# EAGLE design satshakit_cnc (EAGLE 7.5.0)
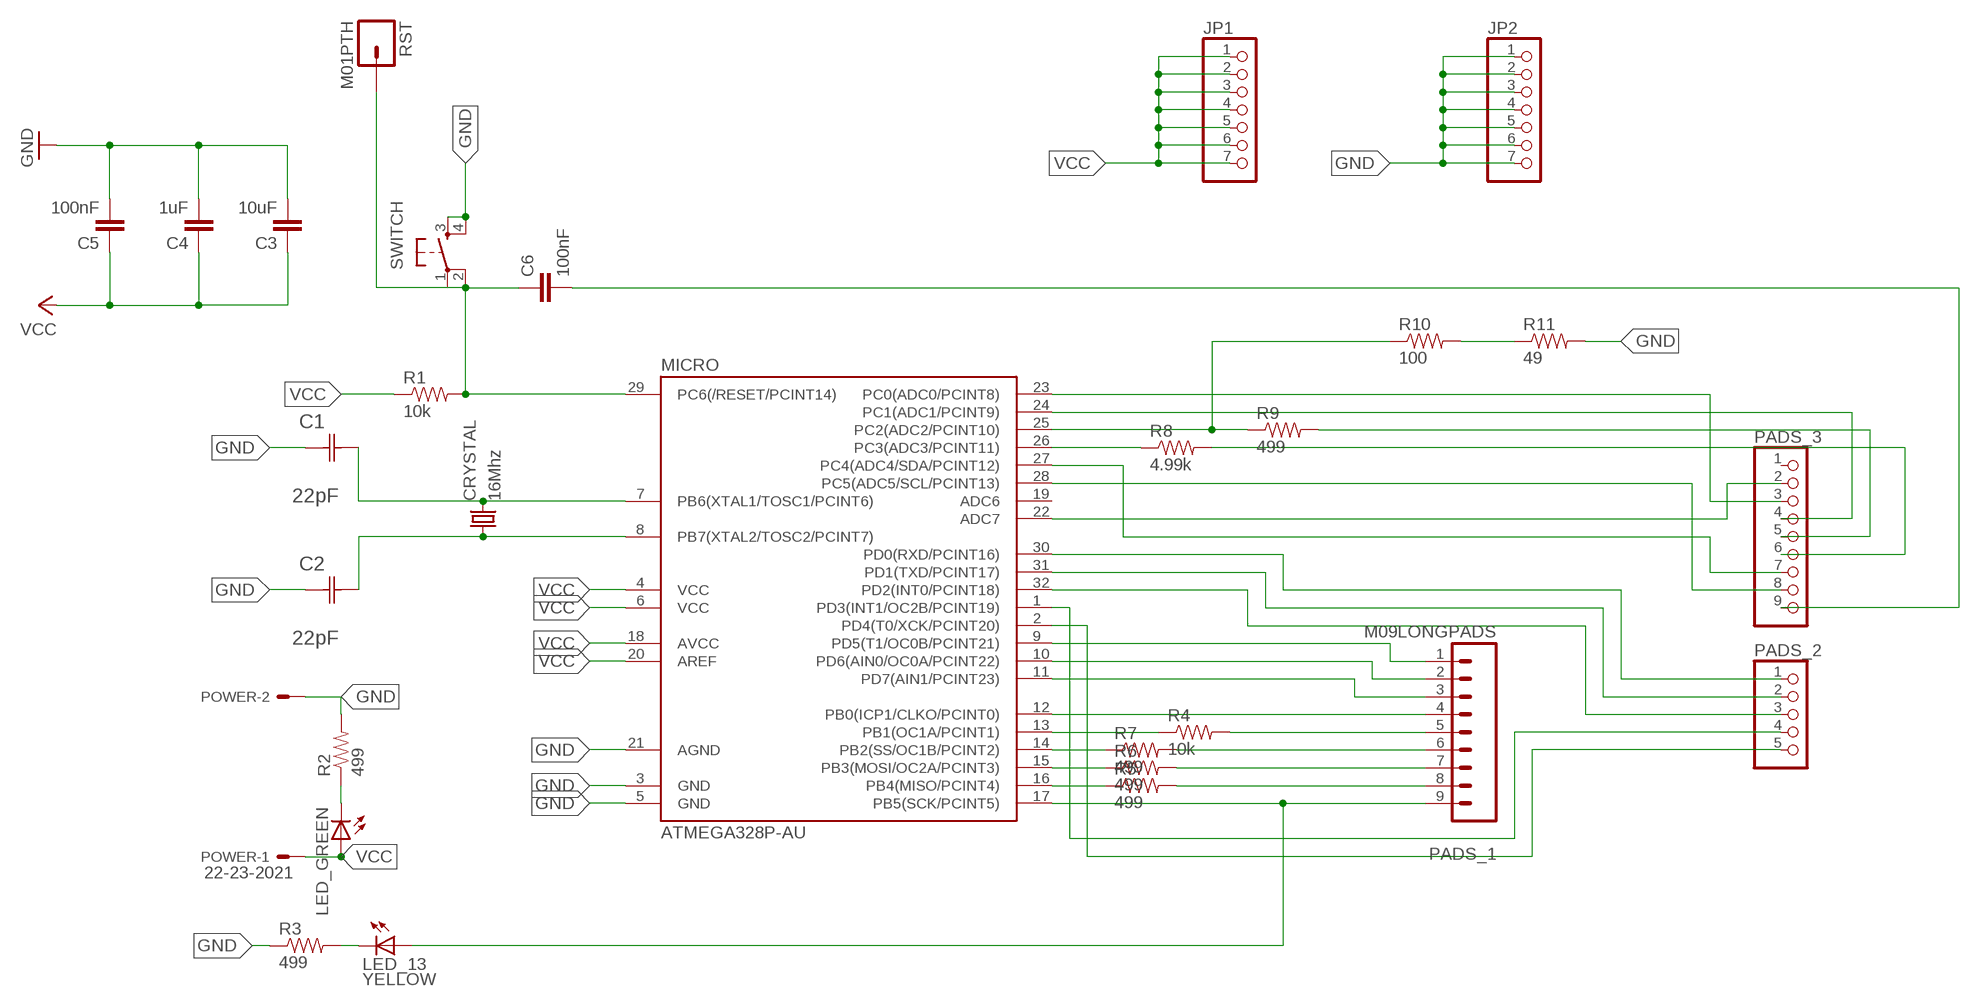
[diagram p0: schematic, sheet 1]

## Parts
C1  22pF  0612ZC225MAT2A  [CAPC3216X178N]
C2  22pF  0612ZC225MAT2A  [CAPC3216X178N]
C3  10uF  CAP1206  [1206]
C4  1uF  CAP1206  [1206]
C5  100nF  CAP1206  [1206]
C6  100nF  CAP1206  [1206]
CRYSTAL  16Mhz  CSM-7X-DU  [CSM-7X-DU]
JP1  PINHD-1X7  [1X07]
JP2  PINHD-1X7  [1X07]
LED_13  YELLOW  LED1206  [1206]
LED_GREEN  LED1206  [1206]
MICRO  ATMEGA328P-AU  ATMEGA48/88/168-AU  [TQFP32-08]
PADS_1  M09LONGPADS  [1X09_LONGPADS]
PADS_2  PINHD-1X5  [1X05]
PADS_3  PINHD-1X9  [1X09]
POWER  22-23-2021  [22-23-2021]
R1  10k  RESISTOR1206  [1206]
R2  499  RESISTOR1206  [1206]
R3  499  RESISTOR1206  [1206]
R4  10k  RESISTOR1206  [1206]
R5  499  RESISTOR1206  [1206]
R6  499  RESISTOR1206  [1206]
R7  499  RESISTOR1206  [1206]
R8  4.99k  RESISTOR1206  [1206]
R9  499  RESISTOR1206  [1206]
R10  100  RESISTOR1206  [1206]
R11  49  RESISTOR1206  [1206]
RST  M01PTH  [1X01]
SWITCH  6MM_SWITCH6MM_SWITCH  [6MM_SWITCH]

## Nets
GND: C1.1(C1) C2.1(C1) C3.2 C4.2 C5.2 JP2.1 JP2.2 JP2.3 JP2.4 JP2.5 JP2.6 JP2.7 MICRO.3(GND) MICRO.5(GND) MICRO.21(AGND) POWER.2 R2.2 R3.1 R11.2 SWITCH.3(S) SWITCH.4(S1)
N$1: MICRO.9(PD5(T1/OC0B/PCINT21)) PADS_1.1
N$2: C1.2(C2) CRYSTAL.2 MICRO.7(PB6(XTAL1/TOSC1/PCINT6))
N$3: C6.2 PADS_3.9
N$4: MICRO.10(PD6(AIN0/OC0A/PCINT22)) PADS_1.2
N$5: MICRO.11(PD7(AIN1/PCINT23)) PADS_1.3
N$6: MICRO.12(PB0(ICP1/CLKO/PCINT0)) PADS_1.4
N$7: MICRO.13(PB1(OC1A/PCINT1)) R4.1
N$8: MICRO.14(PB2(SS/OC1B/PCINT2)) R7.1
N$9: C2.2(C2) CRYSTAL.1 MICRO.8(PB7(XTAL2/TOSC2/PCINT7))
N$10: MICRO.15(PB3(MOSI/OC2A/PCINT3)) R6.1
N$11: MICRO.16(PB4(MISO/PCINT4)) R5.1
N$12: LED_13.1(A) MICRO.17(PB5(SCK/PCINT5)) PADS_1.9
N$13: PADS_1.6 R7.2
N$14: MICRO.22(ADC7) PADS_3.2
N$15: MICRO.23(PC0(ADC0/PCINT8)) PADS_3.3
N$16: MICRO.24(PC1(ADC1/PCINT9)) PADS_3.4
N$17: PADS_3.5 R9.2
N$18: PADS_3.6 R8.2
N$19: MICRO.27(PC4(ADC4/SDA/PCINT12)) PADS_3.7
N$20: MICRO.30(PD0(RXD/PCINT16)) PADS_2.1
N$21: MICRO.31(PD1(TXD/PCINT17)) PADS_2.2
N$22: MICRO.32(PD2(INT0/PCINT18)) PADS_2.3
N$23: MICRO.1(PD3(INT1/OC2B/PCINT19)) PADS_2.4
N$24: MICRO.2(PD4(T0/XCK/PCINT20)) PADS_2.5
N$25: MICRO.28(PC5(ADC5/SCL/PCINT13)) PADS_3.8
N$26: LED_GREEN.2(C) R2.1
N$27: LED_13.2(C) R3.2
N$28: C6.1 MICRO.29(PC6(/RESET/PCINT14)) R1.2 RST.1 SWITCH.1(P) SWITCH.2(P1)
N$30: PADS_1.7 R6.2
N$31: PADS_1.8 R5.2
N$32: PADS_1.5 R4.2
N$33: MICRO.26(PC3(ADC3/PCINT11)) R8.1
N$34: MICRO.25(PC2(ADC2/PCINT10)) R9.1 R10.1
N$35: R10.2 R11.1
VCC: C3.1 C4.1 C5.1 JP1.1 JP1.2 JP1.3 JP1.4 JP1.5 JP1.6 JP1.7 LED_GREEN.1(A) MICRO.4(VCC) MICRO.6(VCC) MICRO.18(AVCC) MICRO.20(AREF) POWER.1 R1.1
Unconnected: MICRO.19(ADC6) PADS_3.1

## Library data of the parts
C1 C2 = AVX_By_element14_Batch_1:0612ZC225MAT2A: Capacitor 1206; MPN: 0612ZC225MAT2A; OC_FARNELL: -; OC_NEWARK: 12N3209; SUPPLIER: AVX; TOLERANCE: ±20%; VALUE: 2.2µF; VOLTAGERATING: 10V
C3-C6 = 01_SparkFun:CAP: Capacitor
CRYSTAL = 01_FAB_Hello:CSM-7X-DU: SMD CRYSTAL; OC_FARNELL: unknown; OC_NEWARK: unknown
JP1 JP2 = pinhead:PINHD-1X7: PIN HEADER
LED_13 LED_GREEN = 01_FAB_Hello:LED
MICRO = atmega8:ATMEGA48/88/168
PADS_1 = 01_SparkFun:M09: Header 9 Standard 9-pin 0.1" header. Use with straight break away headers (SKU : PRT-00116), right angle break away headers (PRT-00553), swiss pins (PRT-00743), machine pins (PRT-00117), and female headers (PRT-00115).
PADS_2 = pinhead:PINHD-1X5: PIN HEADER
PADS_3 = pinhead:PINHD-1X9: PIN HEADER
POWER = con-molex:22-23-2021: .100" (2.54mm) Center Header - 2 Pin; MF: MOLEX; MPN: 22-23-2021; OC_FARNELL: 1462926; OC_NEWARK: 25C3832
R1-R11 = 01_SparkFun:RESISTOR: Resistor
RST = 01_SparkFun:M01: Header 1
SWITCH = 01_FAB_Hello:6MM_SWITCH: OMRON SWITCH

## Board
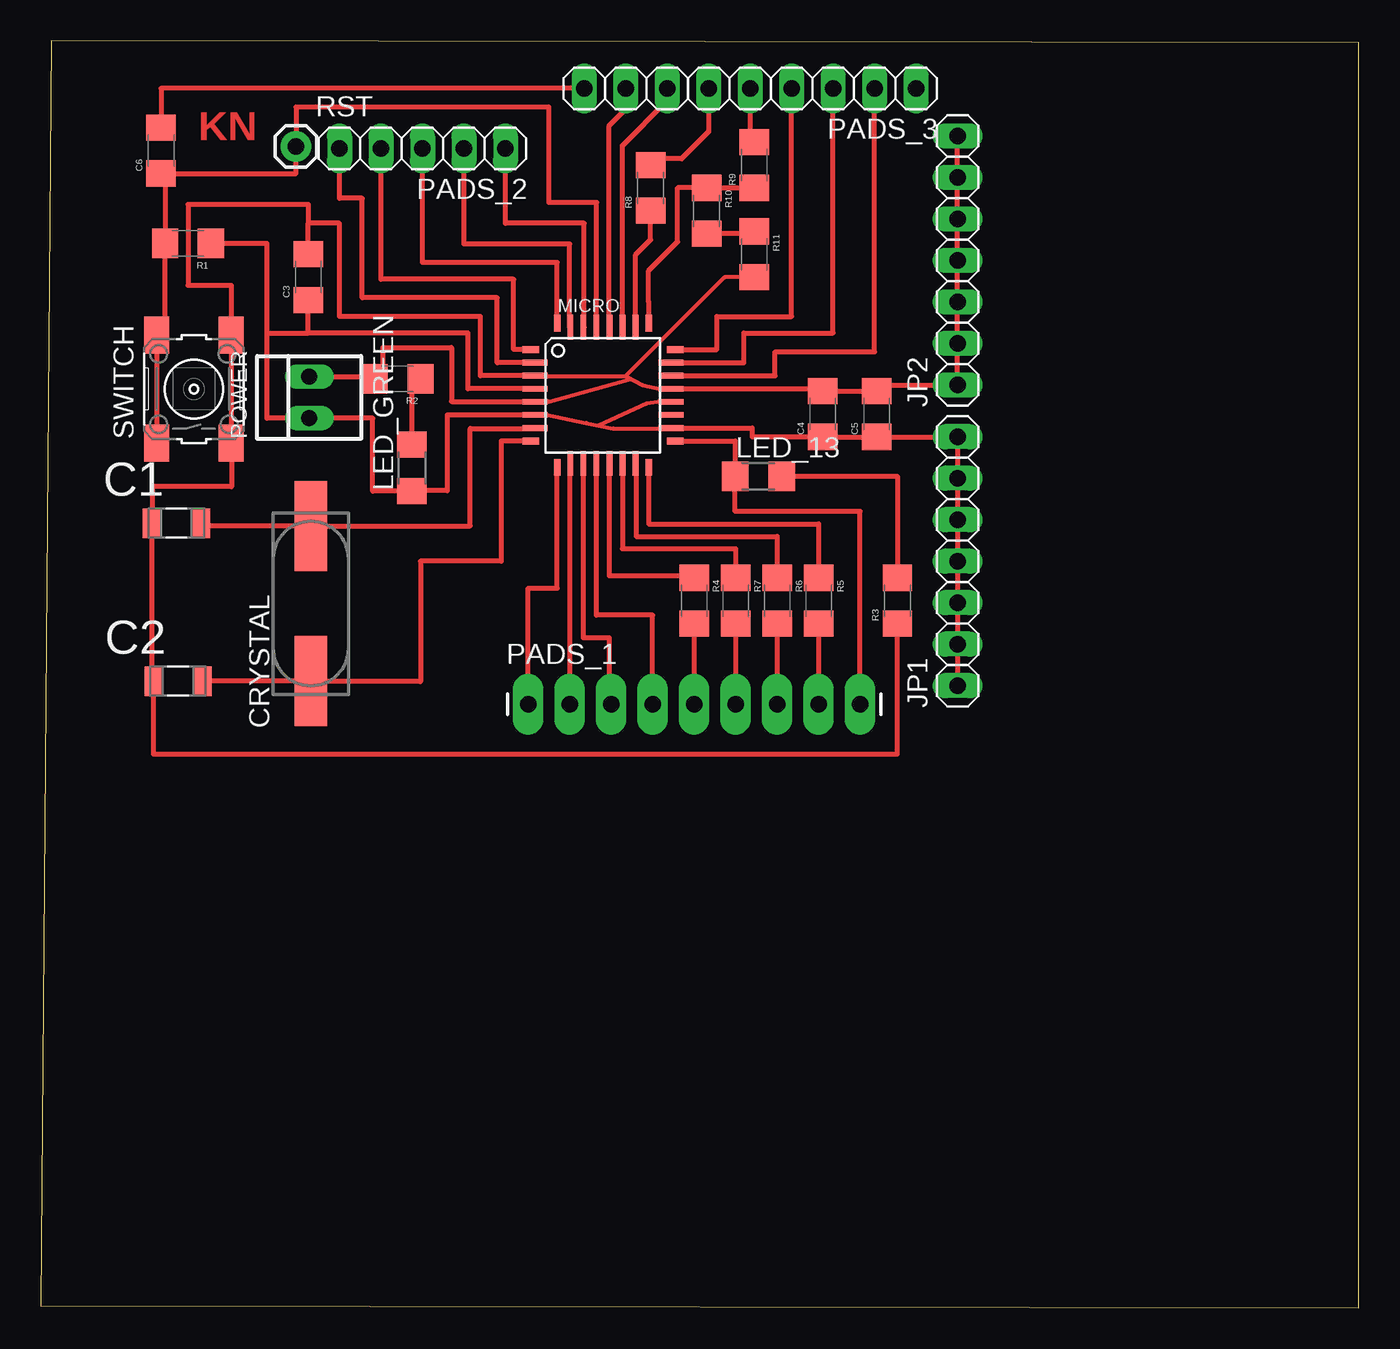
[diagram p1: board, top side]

Size 80.7 x 77.59 mm. Coordinates in mm from the lower left corner, seen from the top.
Outline: 0,0.13 80.7,0 80.7,77.46 0.63,77.59 0,0.13
Copper layers (1*16): Top 0.035mm / dielectric 1.5mm / Bottom 0.035mm
Design rules "default": minimum track width 10mil, minimum drill 24mil, track to track 8mil, track to pad 8mil, pad to pad 8mil, via to via 8mil, smd to smd 8mil, copper to edge 40mil, drill to drill 8mil, minimum pad ring 10mil, minimum via ring 8mil, stop-mask expansion 4mil, vias tented up to drill 0mil, thermal gap 10mil

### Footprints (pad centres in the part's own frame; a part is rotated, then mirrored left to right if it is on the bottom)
CAPC3216X178N = smd 1.118 x 1.803: 1 -1.499,0; 2 1.499,0
1206 = smd 1.6 x 1.8: 1 -1.4,0; 2 1.4,0
CSM-7X-DU = smd 5.5 x 2: 1 -4.75,0; 2 4.75,0
1X07 = drill 1.016 long: 1 -7.62,0; 2 -5.08,0; 3 -2.54,0; 4 0,0; 5 2.54,0; 6 5.08,0; 7 7.62,0
1206' = smd 1.6 x 1.803: 1 -1.422,0; 2 1.422,0
TQFP32-08 = smd 1.016 x 0.406: 1 -4.42,2.8; 8 -4.42,-2.8; 17 4.42,-2.8; 24 4.42,2.8 | smd 1.524 x 0.356: 2 -4.166,2; 3 -4.166,1.2; 4 -4.166,0.4; 5 -4.166,-0.4; 6 -4.166,-1.2; 7 -4.166,-2; 18 4.166,-2; 19 4.166,-1.2; 20 4.166,-0.4; 21 4.166,0.4; 22 4.166,1.2; 23 4.166,2 | smd 0.406 x 1.016: 9 -2.8,-4.42; 16 2.8,-4.42; 25 2.8,4.42; 32 -2.8,4.42 | smd 0.356 x 1.524: 10 -2,-4.166; 11 -1.2,-4.166; 12 -0.4,-4.166; 13 0.4,-4.166; 14 1.2,-4.166; 15 2,-4.166; 26 2,4.166; 27 1.2,4.166; 28 0.4,4.166; 29 -0.4,4.166; 30 -1.2,4.166; 31 -2,4.166
1X09_LONGPADS = drill 1.016 pad 1.88 long: 1 0,0; 2 2.54,0; 3 5.08,0; 4 7.62,0; 5 10.16,0; 6 12.7,0; 7 15.24,0; 8 17.78,0; 9 20.32,0
1X05 = drill 1.016 long: 1 -5.08,0; 2 -2.54,0; 3 0,0; 4 2.54,0; 5 5.08,0
1X09 = drill 1.016 long: 1 -10.16,0; 2 -7.62,0; 3 -5.08,0; 4 -2.54,0; 5 0,0; 6 2.54,0; 7 5.08,0; 8 7.62,0; 9 10.16,0
22-23-2021 = drill 1 long: 1 -1.27,0; 2 1.27,0
1X01 = drill 1.016 pad 1.88: 1 0,0
6MM_SWITCH = smd 2.286 x 1.524: 1 -3.302,2.286; 2 3.302,2.286; 3 -3.302,-2.286; 4 3.302,-2.286

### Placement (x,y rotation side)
C1  8.31,48.06 0 top
C2  8.41,38.38 0 top
C3  16.38,63.12 90 top
C4  47.88,54.74 90 top
C5  51.18,54.74 90 top
C6  7.37,70.87 90 top
CRYSTAL  16.54,43.13 90 top
JP1  56.13,45.72 90 top
JP2  56.13,64.14 90 top
LED_13  YELLOW  [1206']  43.94,50.93 0 top
LED_GREEN  [1206']  22.73,51.44 90 top
MICRO  34.42,55.88 0 top
PADS_1  29.84,36.96 0 top
PADS_2  23.37,70.99 180 top
PADS_3  43.43,74.68 180 top
POWER  16.43,55.75 90 top
R1  9.02,65.18 180 top
R2  21.84,56.9 180 top
R3  52.45,43.31 90 top
R4  40.01,43.31 270 top
R5  47.62,43.31 270 top
R6  45.09,43.31 270 top
R7  42.55,43.31 270 top
R8  37.34,68.58 90 top
R9  43.69,69.98 90 top
R10  40.77,67.18 270 top
R11  43.69,64.52 270 top
RST  15.62,71.12 0 top
SWITCH  9.37,56.26 90 top

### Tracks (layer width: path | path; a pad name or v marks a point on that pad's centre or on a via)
GND
  Top 0.254: MICRO.3 30.28,57.05 35.8,57.05 | 35.8,57.05 36.83,56.52 37.97,56.26 | 30.86,55.5 31.12,55.5 35.99,56.84 | 35.99,56.84 36.13,56.88 | 35.8,57.05 35.99,56.84 | 35.8,57.05 41.87,63.12 R11.2
  Top 0.305: MICRO.5 | MICRO.21 | C1.1 6.81,38.38 C2.1 6.91,33.91 52.45,33.91 R3.1 | C1.1 6.73,48.06 | MICRO.5 30.25,55.5 25.15,55.5 25.15,58.8 20.95,58.8 20.95,56.77 R2.2 20.95,57.02 POWER.2 | C1.1 6.86,48.06 6.86,50.29 11.68,50.29 11.68,52.96 | MICRO.21 47.88,56.28 C4.2 C5.2 | 30.86,55.5 MICRO.5 | MICRO.21 37.97,56.26 | MICRO.3 26.92,57.08 26.92,60.71 18.29,60.71 18.29,66.42 16.38,66.42 | C3.2 16.38,66.42 | SWITCH.3 11.68,52.96 | 11.68,52.96 11.68,58.93 11.66,58.93 SWITCH.4 11.68,59.56 11.68,62.61 9.02,62.61 9.02,67.56 16.38,67.56 16.38,66.42 | 51.18,56.52 JP2.1 JP2.2 JP2.3 JP2.4 JP2.5 JP2.6 JP2.7
  Top 0.406: 51.18,56.52 C5.2
N$1
  Top 0.305: PADS_1.1 29.84,44.07 31.62,44.07 MICRO.9
N$2
  Top 0.305: 9.8,47.88 C1.2 9.8,47.88 | MICRO.7 30.25,53.85 26.29,53.85 26.29,47.88 CRYSTAL.2 9.8,47.88
N$3
  Top 0.305: PADS_3.9 7.37,74.68 C6.2
N$4
  Top 0.305: PADS_1.2 32.42,40.51 MICRO.10
N$5
  Top 0.305: MICRO.11 33.22,41.02 34.8,41.02 34.8,37.59 34.92,37.59 PADS_1.3
N$6
  Top 0.305: 34.04,51.71 MICRO.12 34.02,42.42 37.46,42.42 PADS_1.4
N$7
  Top 0.305: MICRO.13 34.8,51.71 34.8,44.83 40.01,44.83 R4.1
N$8
  Top 0.305: MICRO.14 35.62,46.48 42.55,46.48 R7.1
N$9
  Top 0.305: 9.91,38.35 C2.2 | MICRO.8 28.19,53.09 28.19,45.72 23.24,45.72 23.24,38.35 16.54,38.35 CRYSTAL.1 C2.2 | C2.2
N$10
  Top 0.305: MICRO.15 36.45,51.71 36.45,47.24 45.09,47.24 R6.1
N$11
  Top 0.305: MICRO.16 37.21,48.01 47.62,48.01 R5.1
N$12
  Top 0.305: PADS_1.9 50.16,48.77 42.52,48.77 LED_13.1 42.52,53.08 MICRO.17
N$13
  Top 0.305: R7.2 PADS_1.6
N$14
  Top 0.305: MICRO.22 44.96,57.08 44.96,58.55 51.05,58.55 PADS_3.2
N$15
  Top 0.305: MICRO.23 43.05,57.88 43.05,59.69 48.51,59.69 PADS_3.3
N$16
  Top 0.305: MICRO.24 41.4,58.68 41.4,60.71 45.97,60.71 PADS_3.4
N$17
  Top 0.305: PADS_3.5 43.43,71.38 R9.2
N$18
  Top 0.305: PADS_3.6 40.89,72.01 39.24,70.36 37.72,70.36 R8.2
N$19
  Top 0.305: MICRO.27 35.62,71.18 38.35,73.91 PADS_3.7
N$20
  Top 0.305: MICRO.30 33.27,60.05 33.27,66.42 28.45,66.42 PADS_2.1
N$21
  Top 0.305: MICRO.31 32.38,60.05 32.38,65.15 25.91,65.15 PADS_2.2
N$22
  Top 0.305: MICRO.32 31.62,64.01 23.37,64.01 PADS_2.3
N$23
  Top 0.305: MICRO.1 28.96,58.68 28.96,62.99 20.83,62.99 PADS_2.4
N$24
  Top 0.305: MICRO.2 27.94,57.88 27.94,61.85 19.69,61.85 19.69,67.94 18.29,67.94 PADS_2.5
N$25
  Top 0.305: MICRO.28 34.8,60.05 34.8,72.39 35.69,73.28 35.69,74.55 PADS_3.8
N$26
  Top 0.305: 23.62,56.64 R2.1 23.24,56.52 22.73,56.52 LED_GREEN.2
N$27
  Top 0.305: LED_13.2 52.45,50.93 R3.2
N$28
  Top 0.305: MICRO.29 34.04,60.05 34.04,67.69 31.12,67.69 31.12,73.53 15.62,73.53 RST.1 15.62,69.47 7.62,69.47 | R1.2 7.36,65.18 | R1.2 7.62,59.56 SWITCH.2 SWITCH.1 | C6.1 7.62,69.47 | 7.62,69.47 R1.2
N$30
  Top 0.305: R6.2 PADS_1.7
N$31
  Top 0.305: R5.2 PADS_1.8
N$32
  Top 0.305: R4.2 PADS_1.5
N$33
  Top 0.305: MICRO.26 36.42,64.48 37.34,65.41 R8.1
N$34
  Top 0.305: R9.1 R10.1 38.99,68.58 38.99,65.28 37.21,63.5 37.21,61.59 37.22,61.59 MICRO.25
N$35
  Top 0.305: 40.77,65.92 R10.2 43.69,65.78 R11.1
VCC
  Top 0.254: 30.94,54.69 33.39,54.19 34.15,54.03 | 34.15,54.03 35.05,53.85 38.58,53.85 | MICRO.20 37.97,55.48 37.97,55.5 37.08,55.37 34.15,54.03
  Top 0.305: MICRO.18 | MICRO.20 37.97,55.5 | MICRO.4 26.16,56.28 26.16,59.69 16.38,59.69 | 13.84,59.69 13.84,65.18 R1.1 | 13.84,59.69 13.84,54.48 POWER.1 20.32,54.48 20.32,50.01 LED_GREEN.1 22.73,50.04 24.89,50.04 24.89,54.68 MICRO.6 30.94,54.69 | 38.58,53.85 MICRO.18 | MICRO.18 43.56,53.88 43.56,53.34 C4.1 C5.1 JP1.7 JP1.6 JP1.5 JP1.4 JP1.3 JP1.2 JP1.1 | 13.84,59.69 16.38,59.69 | 16.38,59.69 C3.1 16.76,61.72 16.76,61.47
  Top 0.406: 57.28,53.34 JP1.7

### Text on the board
Top: KN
